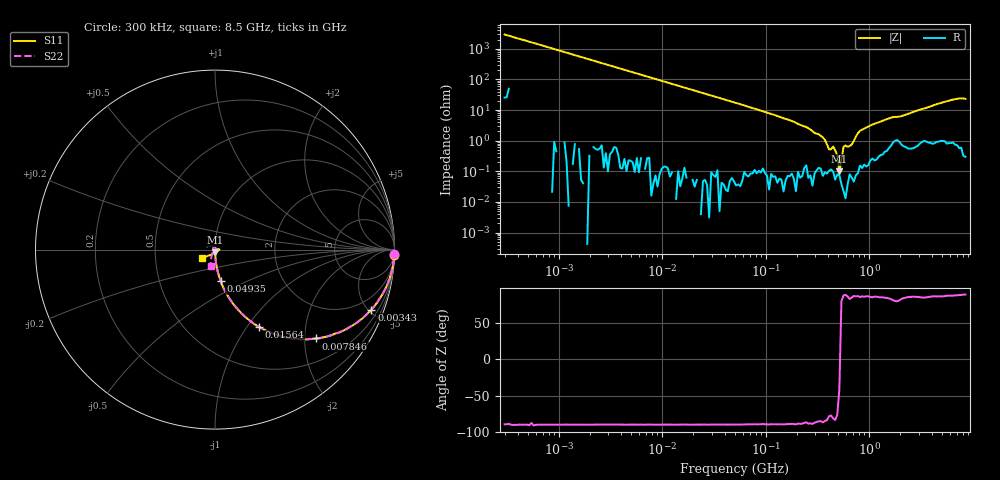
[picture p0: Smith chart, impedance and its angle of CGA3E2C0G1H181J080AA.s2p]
! S-parameter Generated by TDK Corporation
! Copyright(C) 2015 TDK Corporation.
! All Rights Reserved.
! TDK P/N: CGA3E2C0G1H181J080AA (Multilayer Ceramic Chip Capacitors)
! Property: C=180pF
! Size(LxWxT): 1.6x0.8x0.8mm, 0.063x0.031x0.031inches
! Model Type: s2p (Touchstone File Format Version 1.0)
! Frequency: DC=Yes Start=0.3MHz Stop=8500MHz 225points Log-sweep
! Note:
! Model Generated on Jun. 23, 2015
! Hash(MD5):
! Port Assignments:
!  1 ---| |--- 2
! Applicable Conditions:
!  Temperature = 25 degC
!  DC Bias Voltage = 0 V
!  Small Signal Operation
! Terms and conditions regarding TDK Simulation Models
! (1)This simulation model is being provided solely for informational purposes. Please refer to the specifications of the products in terms of detailed characteristics of such products.
! (2)In no event shall TDK Corporation of any of its subsidiaries be liable for any loss or damage arising, directly or indirectly,
!  From any information contained in this simulation model, including, but not limited to loss or damages arising from any inaccuracies, omissions or errors in connection with such information.
! (3)Any and all copyrights on this simulation model are owned by TDK Corporation.
!  Duplication or redistribution of this simulation model without prior written permission from TDK Corporation is prohibited.
! (4)This simulation model is subject to any modification or change without any prior notice.
! (5)Neither TDK Corporation nor any of its subsidiaries shall make any warranty, express or implied,
!  Including but not limited to the correctness, implied warranties of merchantability and fitness for a particular purpose with respect to this simulation models.
! (6)The use of this simulation model shall be deemed to have consented to the terms and conditions hereof.
# MHz S MA R 50
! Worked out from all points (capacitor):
!   224 points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, 300 kHz to 8.5 GHz, reference 50 ohm
!   read as one part in series: C = 179 pF near 314.1 kHz
!   lowest |Z| = 99.1 mohm at 514.7 MHz (marker M1)
!   series resonance near 520.3 MHz, so ESL is about 520 pH
!   S11 on the Smith chart (normalised r, x): 300 kHz: 1, -66; 3.43 MHz: 1.01, -5.22; 7.846 MHz: 1.00, -2.28; 15.64 MHz: 1.00, -1.14; 49.35 MHz: 1.00, -0.36; 8.5 GHz: 0.86, -0.08
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0.3  0.9994 -1.7  0.03381 87.9  0.03381 88.9  0.9994 -1.5
1.72111  0.9817 -10.9  0.1896 79.1  0.189 79.1  0.9812 -10.9
3.429973  0.9331 -21.0  0.3585 68.9  0.3584 69.0  0.9329 -21.0
7.846373  0.7505 -41.2  0.6598 48.7  0.6599 48.6  0.7506 -41.3
9.430415  0.6874 -46.6  0.7261 43.4  0.7261 43.4  0.6873 -46.6
15.63691  0.496 -60.3  0.8681 29.7  0.868 29.8  0.4961 -60.3
49.35002  0.178 -79.9  0.9836 10.0  0.9837 10.1  0.1779 -79.8
51.67171  0.1699 -80.2  0.9847 9.6  0.9852 9.5  0.1698 -80.3
283.1228  0.02943 -87.9  0.9994 0.7  0.9989 0.7  0.02894 -89.8
514.6664  0.0148 -89.4  0.9985 -0.8  0.9981 -0.8  0.0149 -92.8
678.1388  0.01224 -85.2  0.9981 -1.5  0.9985 -1.5  0.0113 -102.4
1124.446  0.004363 -102.2  0.9967 -4.4  0.9973 -4.4  0.006812 -62.8
1551.304  0.004351 -57.0  0.9929 -6.3  0.9928 -6.3  0.007161 -40.0
1864.484  0.01172 -57.1  0.9878 -7.4  0.9882 -7.3  0.01452 -51.6
2044.041  0.01297 -75.9  0.9909 -8.0  0.991 -7.9  0.01539 -69.0
3389.298  0.0117 -49.7  0.9893 -13.4  0.9882 -13.5  0.01139 -60.0
4265.177  0.01081 -2.7  0.9896 -16.9  0.9919 -17.0  0.004366 16.1
4675.929  0.01499 7.4  0.9902 -18.8  0.9888 -18.6  0.008339 39.5
6450.987  0.02505 -0.8  0.9883 -25.4  0.9878 -25.5  0.0135 112.4
7404.957  0.01389 -46.5  0.9899 -29.2  0.9876 -29.1  0.01256 -165.6
7753.325  0.02022 -100.4  0.9867 -30.4  0.9907 -30.4  0.02501 -126.5
8500  0.08516 -147.1  0.9845 -33.3  0.9874 -33.2  0.09489 -105.2
